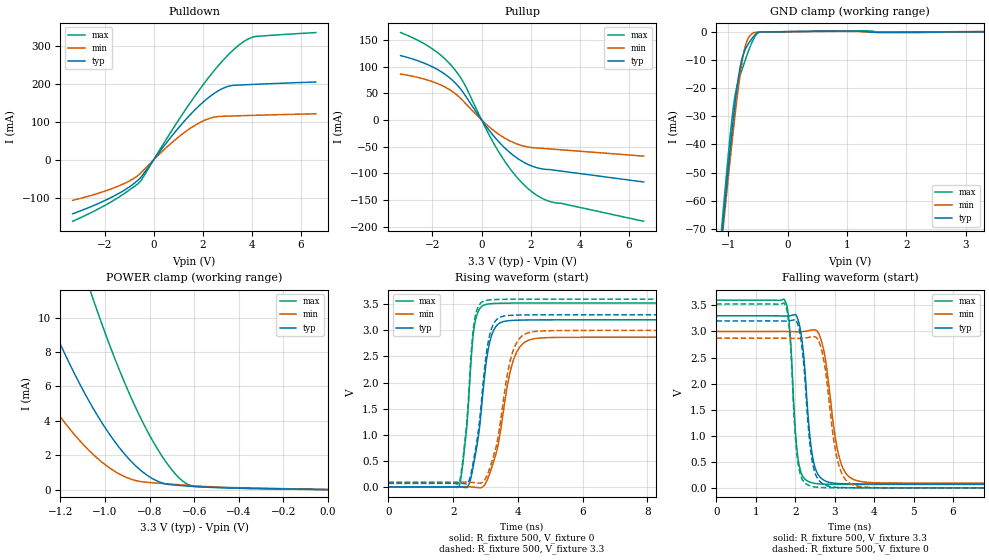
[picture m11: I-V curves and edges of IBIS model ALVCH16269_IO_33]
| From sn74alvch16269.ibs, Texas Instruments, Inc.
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[Model]   ALVCH16269_IO_33
Model_type  3-state
Enable   Active-Low
Vref =   0
Rref =   500
Cref =   50p
Vmeas =   1.5
| variable   typ   min   max
C_comp   7.48pF   6.54pF   8.68pF
| C_pullup   8.62pF   7.24pF   9.62pF
| C_pulldown   8.23pF   7.55pF   9.75pF
| C_tri-state   7.48pF   6.54pF   8.68pF
[Temperature Range]   40   100   -40
| Ambient temperature   25   85   -40
[Voltage range]   3.3   3   3.6
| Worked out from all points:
|   slope of the pulldown table from 0 to 0.495 V, typ, clamps not added: 11.6 ohm
|   slope of the pullup table from 0 to 0.495 V, typ, clamps not added: 16.4 ohm
|   GND clamp passes 1 mA (typ) near -0.54 V on its own axis
|   POWER clamp passes 1 mA (typ) near -0.83 V on its own axis
|   rising waveform, R_fixture 500, V_fixture 0: 20-80 % time 370ps typ, 503ps min, 260ps max; typ from 0 V to 3.2 V
|   falling waveform, R_fixture 500, V_fixture 3.3: 20-80 % time 217ps typ, 314ps min, 162ps max; typ from 3.3 V to 0.073 V
|   rising waveform, R_fixture 500, V_fixture 3.3: 20-80 % time 358ps typ, 478ps min, 256ps max; typ from 0.073 V to 3.3 V
|   falling waveform, R_fixture 500, V_fixture 0: 20-80 % time 214ps typ, 301ps min, 161ps max; typ from 3.2 V to 0 V
[GND Clamp]
| ALVCH16269_IO_33
|   Voltage   I(typ)   I(min)   I(max)
-3.3V     -626.1mA   -593.9mA   -656.2mA
-1.105V   -72.21mA   -74.26mA   -68.64mA
-1.085V   -67.66mA   -69.99mA   -63.82mA
-1.065V   -63.15mA   -65.75mA   -59.05mA
-930mV    -34.26mA   -38.26mA   -29.74mA
-875mV    -23.87mA   -27.95mA   -21.52mA
-820mV    -15.22mA   -18.54mA   -16.83mA
-770mV    -9.805mA   -11.26mA   -13.63mA
-705mV    -6.015mA   -4.647mA   -9.614mA
-585mV    -2.03mA    -551.2uA   -3.121mA
-435mV    -124.1uA   -115.2uA   -161.7uA
3.3V      84.91pA    45.15uA    -78.17uA
[POWER Clamp]
| ALVCH16269_IO_33
|   Voltage   I(typ)   I(min)   I(max)
-3.3V     108.3mA    75.72mA    154.7mA
-1.54V    19.83mA    11.72mA    34.08mA
-1.515V   18.88mA    11.07mA    32.71mA
-1.295V   11.27mA    6.013mA    21.48mA
-1.175V   7.75mA     3.8mA      16.03mA
-1.055V   4.768mA    2.064mA    11.15mA
-950mV    2.682mA    1.011mA    7.422mA
-845mV    1.177mA    476.9uA    4.294mA
-745mV    391.9uA    357uA      1.96mA
-655mV    230.6uA    272.9uA    531.9uA
-600mV    180.2uA    224.4uA    185.4uA
-48.03fV  84.91pA    348.9pA    14.73pA
[Pulldown]
| ALVCH16269_IO_33
|   Voltage   I(typ)   I(min)   I(max)
-3.3V     -142.1mA   -106.8mA   -161.9mA
-1.585V   -94.25mA   -73.08mA   -104.9mA
-965mV    -70.21mA   -54.91mA   -78.36mA
-565mV    -49.04mA   -37.02mA   -58.47mA
810mV     68.36mA    49.08mA    84.25mA
1.875V    143.7mA    97.82mA    185.4mA
2.34V     169.1mA    110.4mA    224.9mA
2.755V    186.1mA    114.4mA    256.9mA
3.11V     194.7mA    115.2mA    281.2mA
3.495V    196.8mA    116mA      303.2mA
4.15V     198.8mA    117.2mA    324.7mA
6.6V      204.9mA    121.2mA    335mA
[Pullup]
| ALVCH16269_IO_33
|   Voltage   I(typ)   I(min)   I(max)
-3.3V     120.6mA    86mA       163.7mA
-2.045V   100.4mA    72.43mA    134.4mA
-1.555V   87.58mA    63.14mA    116.9mA
-1.135V   72.05mA    51.44mA    96.79mA
-685mV    47.06mA    32.31mA    66.09mA
200mV     -12.91mA   -8.674mA   -18.61mA
785mV     -45.09mA   -29.53mA   -66.22mA
1.415V    -70.53mA   -44.56mA   -106.2mA
2.045V    -86.43mA   -51.88mA   -134.5mA
2.45V     -91.62mA   -53.18mA   -146.6mA
2.85V     -93.53mA   -54.59mA   -153.8mA
6.6V      -116.3mA   -67.85mA   -190mA
[Ramp]
| ALVCH16269_IO_33
| variable   typ   min   max
dV/dt_r   1.93/3.78E-10   1.73/5.14E-10   2.12/2.64E-10
dV/dt_f   1.95/2.24E-10   1.77/3.29E-10   2.13/1.66E-10
R_load = 500
[Rising Waveform]
| ALVCH16269_IO_33
R_fixture =   500
C_fixture =   0
L_fixture =   0
V_fixture =   0
V_fixture_min = 0
V_fixture_max = 0
|   Time   V(typ)   V(min)   V(max)
0s        96.47pV    2.363nV    80.17pV
2.19ns    3.908mV    44.54uV    22.14mV
2.42ns    -14.67mV   4.147mV    1.138V
2.57ns    228.8mV    -975.9uV   2.567V
2.66ns    524mV      -7.18mV    3.094V
3.135ns   2.787V     265.8mV    3.51V
3.36ns    3.102V     720.3mV    3.519V
3.88ns    3.194V     2.461V     3.525V
4.66ns    3.202V     2.853V     3.526V
50ns      3.203V     2.87V      3.526V
[Falling Waveform]
| ALVCH16269_IO_33
R_fixture =   500
C_fixture =   0
L_fixture =   0
V_fixture =   3.3
V_fixture_min = 3
V_fixture_max = 3.6
|   Time   V(typ)   V(min)   V(max)
0s        3.3V       3V         3.6V
1.735ns   3.296V     3.001V     3.6V
1.87ns    3.302V     2.998V     2.974V
2.02ns    3.316V     2.995V     937.4mV
2.18ns    2.784V     2.997V     237.4mV
2.39ns    873mV      3.024V     105.8mV
2.565ns   276.4mV    2.999V     79.2mV
3.165ns   80.38mV    465.2mV    67.26mV
3.82ns    73.86mV    106.3mV    66.09mV
50ns      72.65mV    89.46mV    65.89mV
[Rising Waveform]
| ALVCH16269_IO_33
R_fixture =   500
C_fixture =   0
L_fixture =   0
V_fixture =   3.3
V_fixture_min = 3
V_fixture_max = 3.6
|   Time   V(typ)   V(min)   V(max)
0s        72.65mV    89.46mV    65.89mV
2.19ns    76.14mV    89.62mV    88.04mV
2.415ns   57.76mV    93.16mV    1.186V
2.57ns    305mV      87.24mV    2.672V
2.66ns    606.7mV    80.87mV    3.192V
3.11ns    2.862V     318.8mV    3.584V
3.35ns    3.212V     829.3mV    3.593V
3.845ns   3.291V     2.596V     3.598V
4.56ns    3.299V     2.982V     3.6V
50ns      3.3V       3V         3.6V
[Falling Waveform]
| ALVCH16269_IO_33
R_fixture =   500
C_fixture =   0
L_fixture =   0
V_fixture =   0
V_fixture_min = 0
V_fixture_max = 0
|   Time   V(typ)   V(min)   V(max)
0s        3.203V     2.87V      3.526V
1.735ns   3.199V     2.871V     3.525V
1.87ns    3.206V     2.868V     2.873V
2.02ns    3.217V     2.866V     834.7mV
2.175ns   2.676V     2.869V     170.9mV
2.38ns    792.4mV    2.893V     38.3mV
2.555ns   197.4mV    2.87V      12.28mV
3.12ns    7.377mV    399.3mV    1.326mV
3.775ns   1.002mV    13.71mV    185.7uV
50ns      354.5nV    568.8nV    223.3nV
